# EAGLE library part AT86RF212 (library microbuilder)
AT86RF212 - Low-Power SPI-based 700/800/900 MHz Transceiver Digikey: AT86RF212-ZU-ND
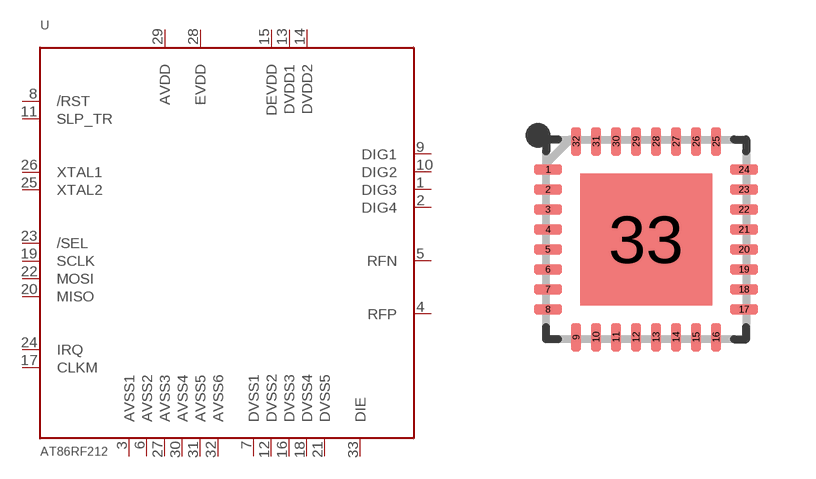
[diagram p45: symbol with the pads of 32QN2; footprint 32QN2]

Designator prefix U

## AT86RF212 (PARTNO: AT86RF212-ZU)  [32QN2]
1  DIG3
2  DIG4
3  AVSS1
4  RFP
5  RFN
6  AVSS2
7  DVSS1
8  /RST
9  DIG1
10  DIG2
11  SLP_TR
12  DVSS2
13  DVDD1
14  DVDD2
15  DEVDD
16  DVSS3
17  CLKM
18  DVSS4
19  SCLK
20  MISO
21  DVSS5
22  MOSI
23  /SEL
24  IRQ
25  XTAL2
26  XTAL1
27  AVSS3
28  EVDD
29  AVDD
30  AVSS4
31  AVSS5
32  AVSS6
33  DIE

## Footprint 32QN2 (pad centres in mm)
32QN2, 32-lead 5.0 x 5.0mm Body, 0.50mm Pitch, Quad Flat No Lead Package (QFN) Sawn
smd 0.7 x 0.25: 1 -2.45,1.75; 2 -2.45,1.25; 3 -2.45,0.75; 4 -2.45,0.25; 5 -2.45,-0.25; 6 -2.45,-0.75; 7 -2.45,-1.25; 8 -2.45,-1.75; 17 2.45,-1.75; 18 2.45,-1.25; 19 2.45,-0.75; 20 2.45,-0.25; 21 2.45,0.25; 22 2.45,0.75; 23 2.45,1.25; 24 2.45,1.75
smd 0.25 x 0.7: 9 -1.75,-2.45; 10 -1.25,-2.45; 11 -0.75,-2.45; 12 -0.25,-2.45; 13 0.25,-2.45; 14 0.75,-2.45; 15 1.25,-2.45; 16 1.75,-2.45; 25 1.75,2.45; 26 1.25,2.45; 27 0.75,2.45; 28 0.25,2.45; 29 -0.25,2.45; 30 -0.75,2.45; 31 -1.25,2.45; 32 -1.75,2.45
smd 3.3 x 3.3: 33 0,0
